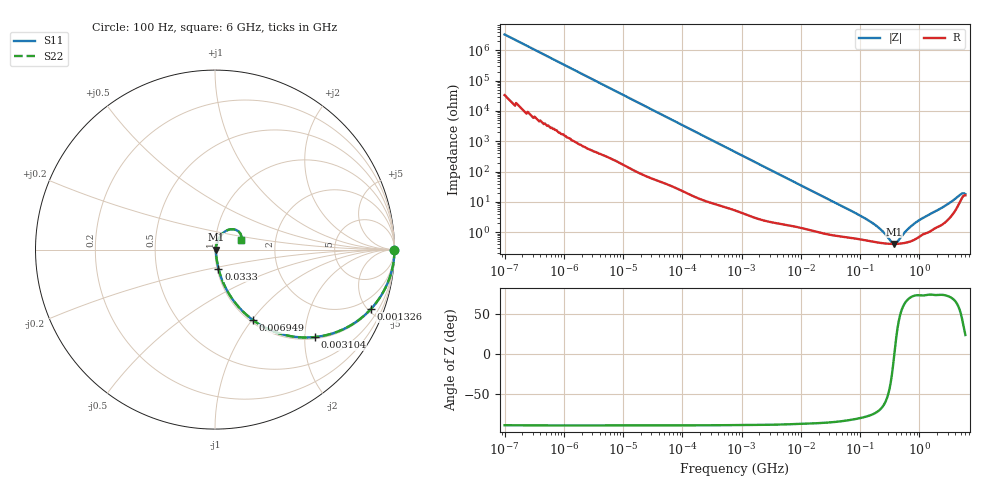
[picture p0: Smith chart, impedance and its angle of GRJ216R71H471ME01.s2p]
!Murata Part Number: GRJ216R71H471ME01
!These Parameters are Measured in Series Mode Connection
!Data Generated on Jun 19, 2026
!  o--ll--o
!Port1  Port2
!  o------o
!Operation Temp=25[degC], DC Bias Voltage=0[V]
!Freq. Start=100[Hz] Stop=6[GHz] 401[Steps]
# Hz S RI R 50
!Freq.(Hz) S11(Real) S11(Imag) S21(Real) S21(Imag) S12(Real) S12(Imag) S22(Real) S22(Imag)
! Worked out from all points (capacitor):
!   401 points, 100 Hz to 6 GHz, reference 50 ohm
!   read as one part in series: C = 473 pF near 109 Hz
!   lowest |Z| = 414 mohm at 373.7 MHz (marker M1)
!   series resonance near 379.4 MHz, so ESL is about 370 pH
!   S11 on the Smith chart (normalised r, x): 100 Hz: open; 1.326 MHz: 1.07, -5.25; 3.104 MHz: 1.04, -2.25; 6.949 MHz: 1.03, -1.01; 33.3 MHz: 1.02, -0.22; 6 GHz: 1.33, +0.15
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100  1 -2.98e-05  3e-07 2.98e-05  3e-07 2.98e-05  1 -2.98e-05
350  1 -0.000104  6e-07 0.000104  6e-07 0.000104  1 -0.000104
2008  1 -0.000592  2.9e-06 0.000592  2.9e-06 0.000592  1 -0.000592
40335  0.9998 -0.0118  0.000206 0.0118  0.000206 0.0118  0.9998 -0.0118
241822  0.9946 -0.0698  0.00543 0.0698  0.00543 0.0698  0.9946 -0.0698
774597  0.9501 -0.2118  0.0499 0.2118  0.0499 0.2118  0.9501 -0.2118
1325623  0.8698 -0.3298  0.1302 0.3298  0.1302 0.3298  0.8698 -0.3298
1983483  0.7521 -0.4242  0.2479 0.4242  0.2479 0.4242  0.7521 -0.4242
3103719  0.558 -0.4871  0.442 0.4871  0.442 0.4871  0.558 -0.4871
6948629  0.2121 -0.3931  0.7879 0.3931  0.7879 0.3931  0.2121 -0.3931
1.555665e7  0.0596 -0.2137  0.9404 0.2137  0.9404 0.2137  0.0596 -0.2137
3.330331e7  0.0193 -0.1053  0.9807 0.1053  0.9807 0.1053  0.0193 -0.1053
1.596157e8  0.00532 -0.0198  0.9947 0.0198  0.9947 0.0198  0.00532 -0.0198
2.283698e8  0.00452 -0.0109  0.9955 0.0109  0.9955 0.0109  0.00452 -0.0109
3.124326e8  0.00416 -0.00408  0.9958 0.00408  0.9958 0.00408  0.00416 -0.00408
3.737127e8  0.00411 -0.000315  0.9959 0.000315  0.9959 0.000315  0.00411 -0.000315
4.274388e8  0.00415 0.00252  0.9959 -0.00252  0.9959 -0.00252  0.00415 0.00252
6.395615e8  0.0048 0.0116  0.9952 -0.0116  0.9952 -0.0116  0.0048 0.0116
9.569533e8  0.00718 0.0226  0.9928 -0.0226  0.9928 -0.0226  0.00718 0.0226
2.931063e9  0.029 0.0742  0.971 -0.0742  0.971 -0.0742  0.029 0.0742
4.796499e9  0.1012 0.1135  0.8988 -0.1135  0.8988 -0.1135  0.1012 0.1135
6e9  0.1456 0.0534  0.8544 -0.0534  0.8544 -0.0534  0.1456 0.0534
